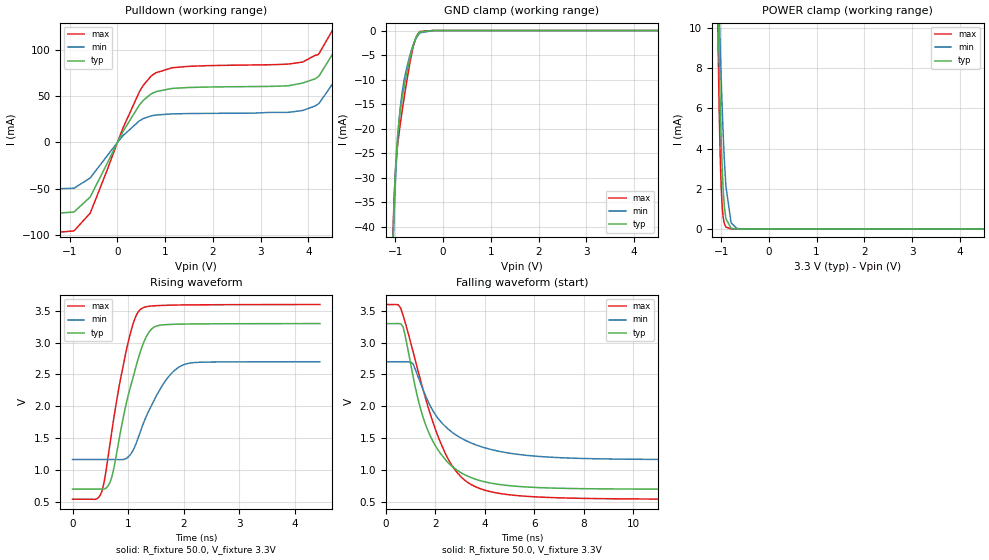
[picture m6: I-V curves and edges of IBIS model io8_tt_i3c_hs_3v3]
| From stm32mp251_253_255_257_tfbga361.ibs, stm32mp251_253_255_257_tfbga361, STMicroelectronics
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[Model]   io8_tt_i3c_hs_3v3
Model_type I/O_open_drain
Polarity   Non-Inverting
Enable   Active-Low
| CAP_THRESHOLD on pad IOTT is "UDTCAPC" :
| Rising=30.0% of vddiov33m   Falling=70.0% of vddiov33m
| C_comp min and max val. don't necessarily correlate with the min and max pvt
| but are the smallest and greatest pad capacitance found.
| var   typ   min   max
C_comp   1.30235pF  1.06404pF  2.26695pF
|C_comp_pulldown   1.30235pF  1.06404pF  2.26695pF
Vinl = 1.35V
Vinh = 1.8V
Vmeas = 1.65V   | Reference voltage for timing measurements
Cref  = 50.0pF   | Timing specification test load capacitance value
Rref  = 1.0MOhm   | Timing specification test load resistance value
Vref  = 1.815V   | Timing specification test load voltage
[Model Spec]
| TIME_THRESHOLD on pin ZIV08M is "CMOS" :
| Rising=50.0% of vddv08m   Falling=50.0% of vddv08m
Vinl 1.08570V 868.70000mV 1.21270V
Vinh 1.55630V 1.26330V 1.71030V
| variable   typ   min   max
[Temperature Range] 25.0 125.0 -40.0
| variable   typ   min   max
[Voltage Range] 3.3V 2.7V 3.6V
| variable   typ   min   max
[POWER Clamp Reference] 3.3V 2.7V 3.6V
| variable   typ   min   max
[GND Clamp Reference] 0V 0V 0V
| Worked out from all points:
|   slope of the pulldown table from 0 to 0.495 V, typ, clamps not added: 11.6 ohm
|   GND clamp passes 1 mA (typ) near -0.55 V on its own axis
|   POWER clamp passes 1 mA (typ) near -0.93 V on its own axis
|   rising waveform, R_fixture 50.0, V_fixture 3.3V: 20-80 % time 407ps typ, 498ps min, 365ps max; typ from 0.695 V to 3.3 V
|   falling waveform, R_fixture 50.0, V_fixture 3.3V: 20-80 % time 1.35ns typ, 1.82ns min, 1.54ns max; typ from 3.3 V to 0.695 V
[POWER Clamp]
-3.3V     1.353A     318.4mA    2.015A
-1.07V    12.07mA    13.62mA    10.38mA
-1.06V    10.79mA    12.67mA    8.742mA
-1.05V    9.57mA     11.75mA    7.25mA
-1.03V    7.34mA     9.996mA    4.745mA
-1V       4.587mA    7.593mA    2.212mA
-980mV    3.182mA    6.169mA    1.235mA
-950mV    1.703mA    4.334mA    479uA
-900mV    514.6uA    2.139mA    90.78uA
-790mV    28.73uA    299.8uA    2.713uA
-670mV    1.278uA    27.48uA    388.8nA
6.6V      0A         0A         0A
[GND Clamp]
-3.3V     -3.772A    -3.743A    -3.788A
-1.05V    -42.34mA   -45.44mA   -41.2mA
-1.04V    -38.9mA    -42mA      -37.88mA
-1.03V    -35.84mA   -38.88mA   -35.06mA
-1V       -28.57mA   -31.07mA   -28.88mA
-970mV    -23.48mA   -25.09mA   -24.97mA
-920mV    -18.07mA   -17.99mA   -20.63mA
-860mV    -13.91mA   -12.68mA   -16.46mA
-770mV    -9.031mA   -7.879mA   -10.78mA
-640mV    -3.394mA   -3.285mA   -3.897mA
-480mV    -254.3uA   -469.3uA   -191.8uA
6.6V      220.4nA    5.137uA    223.2nA
| variable   typ   min   max
[Pullup Reference] 3.3V 2.7V 3.6V
| variable   typ   min   max
[Pulldown Reference] 0V 0V 0V
[Pulldown]
-3.3V     -76.59mA   -50.19mA   -97.29mA
-910mV    -75.37mA   -49.66mA   -95.8mA
-570mV    -59.08mA   -38.48mA   -76.52mA
120mV     12mA       7.376mA    15.98mA
460mV     40.46mA    23.32mA    54.73mA
800mV     54.75mA    29.51mA    75.15mA
1.48V     59.3mA     31.12mA    82.16mA
3.88V     64.18mA    34.44mA    86.87mA
4.22V     71.69mA    42.05mA    95.8mA
4.56V     99.99mA    67.27mA    126.4mA
4.9V      185.2mA    140.4mA    220.4mA
6.6V      1.447A     1.603A     1.41A
[Ramp]
dV/dt_r 1.56183V/406.72674ps 922.56807mV/497.92467ps 1.83752V/364.91769ps
dV/dt_f 1.56279V/1.34494ns 923.47202mV/1.81621ns 1.83839V/1.53379ns
R_load = 50.0
| Removed startup time: 0s 0s 0s  .
| Removed end time: 4.45ns.
[Rising Waveform]
R_fixture   = 50.0
V_fixture   = 3.3V
V_fixture_min = 2.7V
V_fixture_max = 3.6V
0s        695.3mV    1.161V     536mV
525ps     693.6mV    1.161V     654.2mV
700ps     867.1mV    1.161V     1.563V
975ps     2.074V     1.183V     2.908V
1.1ns     2.486V     1.324V     3.322V
1.225ns   2.87V      1.61V      3.524V
1.45ns    3.233V     2.062V     3.577V
1.725ns   3.284V     2.461V     3.587V
2ns       3.291V     2.652V     3.592V
4.45ns    3.298V     2.698V     3.599V
| Removed startup time: 0s 0s 0s  .
| Removed end time: 24.9ns.
[Falling Waveform]
R_fixture   = 50.0
V_fixture   = 3.3V
V_fixture_min = 2.7V
V_fixture_max = 3.6V
0s        3.3V       2.7V       3.6V
500ps     3.301V     2.7V       3.596V
700ps     3.246V     2.7V       3.425V
1.1ns     2.47V      2.667V     2.857V
1.4ns     1.962V     2.363V     2.41V
2ns       1.379V     1.869V     1.639V
2.8ns     1.016V     1.557V     996.6mV
3.9ns     820.9mV    1.358V     691.8mV
8.3ns     702.1mV    1.176V     548.9mV
24.9ns    695.3mV    1.161V     536mV
